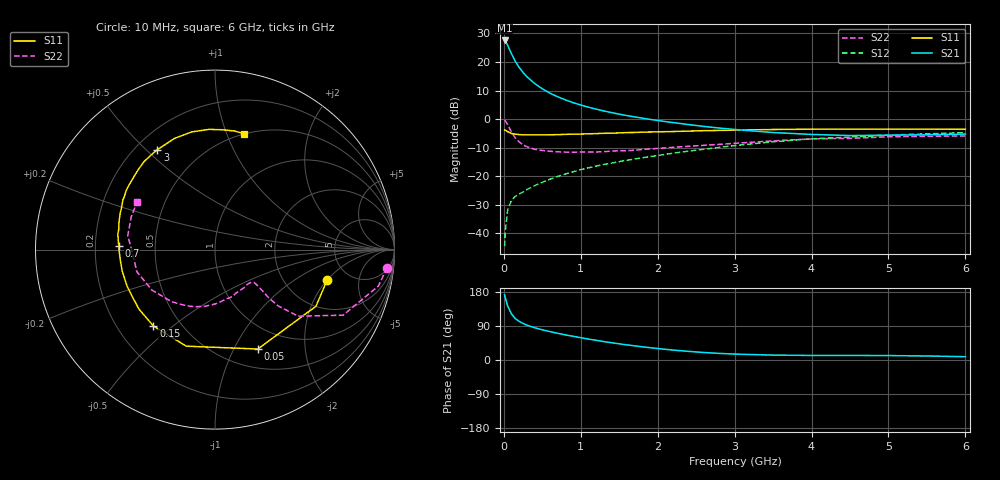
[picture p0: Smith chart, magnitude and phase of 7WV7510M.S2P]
! Infineon Technologies  Discrete & RF Semiconductors
! BFS17W
! Si NPN RF Bipolar Junction Transistor in SOT323
! VCE = 0.75 V  IC = 10 mA
! Common Emitter S-Parameters:  August  1999
# GHz  S  MA  R  50
!  f  S11  S21  S12  S22
! GHz  MAG  ANG  MAG  ANG  MAG  ANG  MAG  ANG
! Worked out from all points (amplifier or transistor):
!   36 points, 10 MHz to 6 GHz, reference 50 ohm
!   highest |S21| = 27.5 dB at 10 MHz (marker M1)
!   |S21| within 3 dB of that: start of sweep to 71.62 MHz
!   unconditionally stable (mu >= 1): 310.2 MHz to end of sweep
!   at 250 MHz: K = 0.90, MSG = 20.9 dB, |S12| = -25.5 dB
!   at 1.4 GHz: K = 1.37, MAG = 5.2 dB, |S12| = -15.4 dB
!   at 6 GHz: K = 1.13, MAG = -2.4 dB, |S12| = -4.7 dB
!   S11 on the Smith chart (normalised r, x): 10 MHz: 3.46, -1.99; 50 MHz: 0.72, -1.25; 150 MHz: 0.35, -0.43; 700 MHz: 0.30, +0.02; 3 GHz: 0.29, +0.54; 6 GHz: 0.50, +1.15
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0.01  0.6479 -14.9  23.84 172.0  0.006 81.0  0.9648 -6.0
0.02  0.645 -29.3  23.19 163.3  0.0114 77.7  0.9324 -12.6
0.05  0.6031 -66.7  19.64 142.3  0.0258 62.0  0.8019 -27.1
0.1  0.5614 -106.6  13.83 121.3  0.0381 50.3  0.5933 -38.7
0.15  0.5466 -128.9  10.23 109.2  0.0448 46.6  0.468 -41.8
0.2  0.5381 -141.8  8.024 101.7  0.0492 47.5  0.3998 -41.9
0.25  0.5301 -150.9  6.556 96.3  0.0532 47.9  0.3546 -41.1
0.3  0.5304 -157.5  5.529 92.0  0.0586 50.2  0.3299 -40.6
0.4  0.5307 -166.8  4.21 85.1  0.0686 52.7  0.2969 -40.1
0.5  0.5305 -173.2  3.4 79.7  0.0787 55.5  0.2841 -40.2
0.6  0.533 -178.0  2.847 74.8  0.0889 56.8  0.2744 -41.4
0.7  0.5367 177.8  2.466 70.5  0.0998 58.0  0.2688 -43.7
0.9  0.5482 170.8  1.946 62.6  0.1201 59.2  0.2639 -49.5
1.1  0.5549 164.7  1.62 55.2  0.1411 59.6  0.2666 -56.6
1.3  0.5662 158.9  1.392 48.6  0.1613 59.3  0.2696 -64.6
1.6  0.5831 151.6  1.155 39.9  0.1908 58.7  0.2813 -76.5
2.2  0.608 137.8  0.872 26.2  0.2534 57.0  0.3219 -100.6
3  0.6428 120.0  0.66 15.6  0.3451 51.4  0.3781 -130.1
3.5  0.6595 109.9  0.584 12.9  0.4032 46.3  0.4174 -147.2
4.5  0.6706 92.8  0.517 12.0  0.4871 34.1  0.4611 -178.3
5.5  0.6695 80.7  0.533 10.6  0.5541 23.5  0.5012 158.6
6  0.6658 75.9  0.549 8.7  0.5815 18.4  0.5093 148.4
